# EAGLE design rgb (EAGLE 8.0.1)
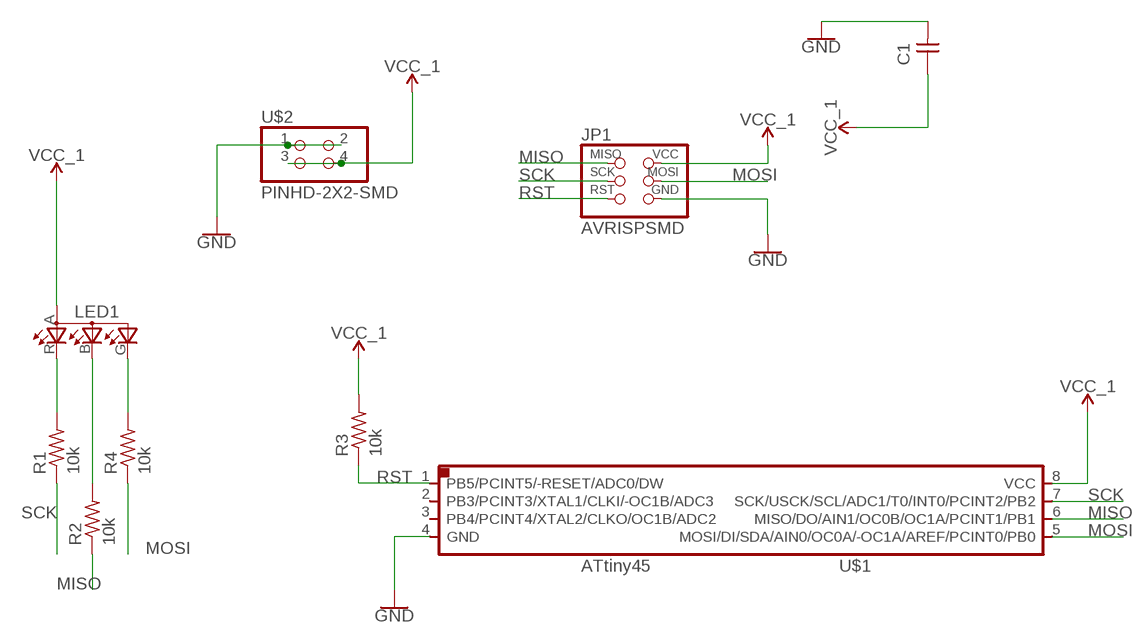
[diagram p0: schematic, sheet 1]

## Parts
C1  CAP-UNPOLARIZEDFAB  [C1206FAB]
JP1  AVRISPSMD  [2X03SMD]
LED1  LEDRGBOLD  [P-LCC-4-3]
R1  10k  RES-US1206  [R1206]
R2  10k  RES-US1206  [R1206]
R3  10k  RES-US1206  [R1206]
R4  10k  RES-US1206  [R1206]
U$1  ATTINY45SI  [SOIC8]
U$2  PINHD-2X2-SMD  [2X02SMD]

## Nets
GND: C1.2 JP1.6(GND) U$1.4(GND) U$2.1 U$2.2
MISO: JP1.1(MISO) R2.1 U$1.6(MISO/DO/AIN1/OC0B/OC1A/PCINT1/PB1)
MOSI: JP1.4(MOSI) R4.1 U$1.5(MOSI/DI/SDA/AIN0/OC0A/-OC1A/AREF/PCINT0/PB0)
N$3: LED1.R(CRED) R1.2
N$4: LED1.B(CBLUE) R2.2
N$5: LED1.G(CGREEN) R4.2
RST: JP1.5(RST) R3.1 U$1.1(PB5/PCINT5/-RESET/ADC0/DW)
SCK: JP1.3(SCK) R1.1 U$1.7(SCK/USCK/SCL/ADC1/T0/INT0/PCINT2/PB2)
VCC_1: C1.1 JP1.2(VCC) LED1.A(A2) R3.2 U$1.8(VCC) U$2.3 U$2.4
Unconnected: U$1.2(PB3/PCINT3/XTAL1/CLKI/-OC1B/ADC3) U$1.3(PB4/PCINT4/XTAL2/CLKO/OC1B/ADC2)

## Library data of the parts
C1 = fab:CAP-UNPOLARIZED
JP1 = fab:AVRISP
LED1 = fab:LEDRGBOLD: OSRAM Hyper Multi TOPLED® Hyper-Bright LED LATB T686 Source: http://www.osram.convergy.de/
R1-R4 = fab:RES-US: Resistor (US Symbol)
U$1 = fab:ATTINY45
U$2 = fab:PINHD-2X2-SMD

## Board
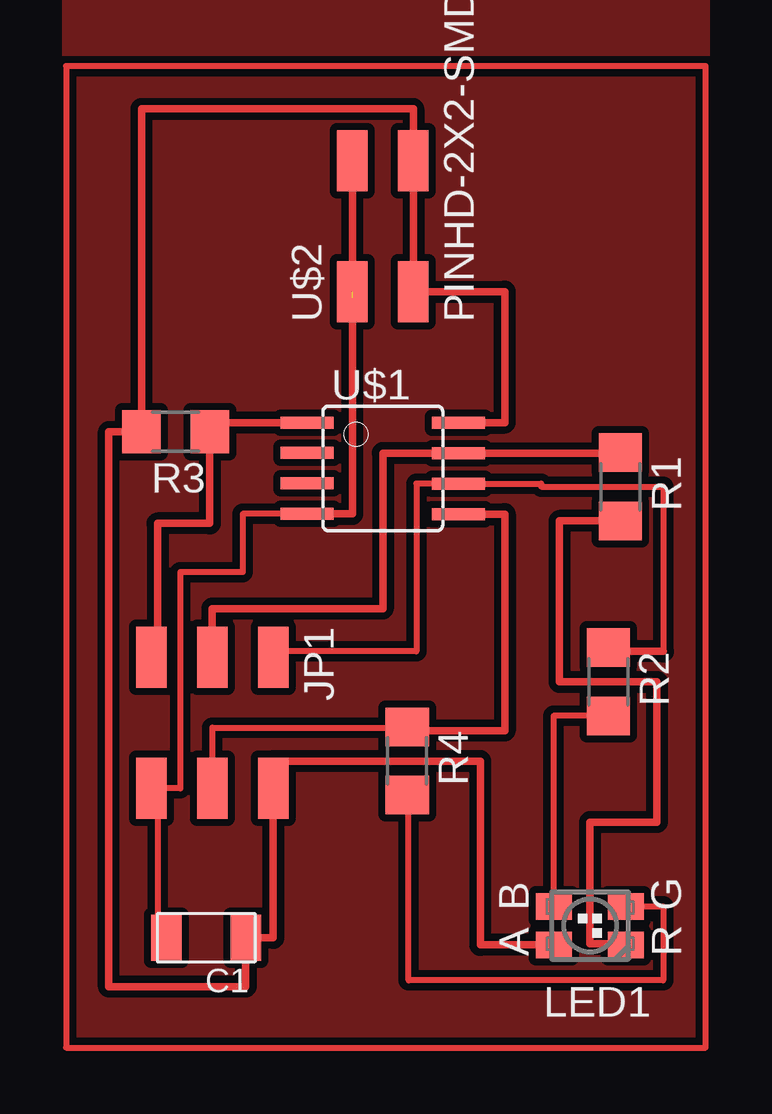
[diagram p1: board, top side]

No outline drawn. Coordinates in mm, seen from the top.
Copper layers (1*16): Top 0.035mm / dielectric 1.5mm / Bottom 0.035mm
Design rules "default *": minimum track width 10mil, minimum drill 24mil, track to track 12mil, track to pad 12mil, pad to pad 12mil, via to via 8mil, smd to smd 8mil, copper to edge 40mil, drill to drill 8mil, minimum pad ring 10mil, minimum via ring 8mil, stop-mask expansion 4mil, vias tented up to drill 0mil, thermal gap 10mil

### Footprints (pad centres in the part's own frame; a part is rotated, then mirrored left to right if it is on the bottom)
C1206FAB = smd 1.27 x 1.905: 1 -1.651,0; 2 1.651,0
2X03SMD = smd 2.54 x 1.27: 1 -2.54,2.54; 2 2.92,2.54; 3 -2.54,0; 4 2.92,0; 5 -2.54,-2.54; 6 2.92,-2.54
P-LCC-4-3 = smd 1.1 x 1.5: A -0.8,1.5; B 0.8,1.5; G 0.8,-1.5; R -0.8,-1.5
R1206 = smd 1.6 x 1.803: 1 -1.422,0; 2 1.422,0
SOIC8 = smd 0.5 x 2.2: 1 -1.905,-3.154; 2 -0.645,-3.154; 3 0.625,-3.154; 4 1.895,-3.154; 5 1.905,3.154; 6 0.635,3.154; 7 -0.635,3.154; 8 -1.905,3.154
2X02SMD = smd 2.54 x 1.27: 1 -2.54,1.27; 2 2.92,1.27; 3 -2.54,-1.27; 4 2.92,-1.27

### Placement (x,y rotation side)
C1  6.1,4.83 180 top
JP1  6.35,13.97 270 top
LED1  22.1,5.33 90 top
R1  23.37,23.62 270 top
R2  22.86,15.49 270 top
R3  4.83,25.91 180 top
R4  14.48,12.19 270 top
U$1  13.46,24.38 270 top
U$2  13.46,34.29 90 top

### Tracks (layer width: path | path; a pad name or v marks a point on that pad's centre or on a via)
_OUTLINES_
  pour Top (isolate 0.12, rank 6): 0.13,0.13 27.05,0.13 27.05,44.27 0.13,44.27
GND  (1 unrouted)
  Top 0.254: C1.2 4.38,5.02 4.06,5.33 4.06,11.05 JP1.6 | 12,32.32 11.68,32.64 | 10.41,22.48 U$1.4 | 9.78,22.48 10.1,22.48 U$1.4 | 4.06,11.37 JP1.6 | JP1.6 5.02,11.05 5.02,20.07 7.62,20.07 7.62,22.49 U$1.4
  Top 0.305: U$1.4 12.19,22.49 12.19,31.5 12,31.5 12,32.32 | U$2.1 U$2.2
MISO
  Top 0.254: 15.81,23.75 U$1.6 | JP1.1 9.14,16.76 14.86,16.76 14.86,23.75 U$1.6 | U$1.6 20.07,23.75 20.07,23.62 25.15,23.62 25.15,16.76
  Top 0.305: 25.15,16.76 22.86,16.76 R2.1
MOSI
  Top 0.254: 14.54,13.91 R4.1 14.22,13.59 6.35,13.59 JP1.4 6.6,11.37 | 16.45,22.48 U$1.5
  Top 0.305: U$1.5 18.54,22.48 18.54,13.46 14.48,13.46 R4.1
N$2
  Top 0.254: 26.92,0.25 26.92,41.15 0.25,41.15 0.25,0.25 26.92,0.25
N$3
  Top 0.305: R1.2 20.83,22.2 20.83,15.49 24.89,15.49 24.89,9.65 22.1,9.65 22.1,4.57 23.6,4.57 LED1.R
N$4
  Top 0.254: LED1.B 20.57,6.29 20.57,14.07 R2.2
  Top 0.305: 22.86,13.91 R2.2
N$5
  Top 0.254: 23.75,5.97 LED1.G 25.15,6.13 25.15,3.05 14.54,3.05 14.54,10.73 R4.2
RST
  Top 0.305: U$1.1 6.25,26.29 R3.1 6.25,22.1 4.06,22.1 4.06,16.51 JP1.5
SCK
  Top 0.254: 15.81,25.02 U$1.7
  Top 0.305: JP1.3 6.35,18.54 13.46,18.54 13.46,25.02 U$1.7 23.37,25.02 R1.1
VCC_1
  Top 0.254: 7.87,5.02 C1.1 7.56,4.7 | JP1.2 8.83,11.05 | 3.43,25.97 R3.2 3.11,25.65
  Top 0.305: U$1.8 18.54,26.29 18.54,31.75 U$2.3 U$2.4 14.73,39.37 3.4,39.37 R3.2 2.03,25.91 2.03,2.79 7.75,2.79 C1.1 8.89,4.83 JP1.2 8.89,12.19 17.53,12.19 17.53,4.53 LED1.A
